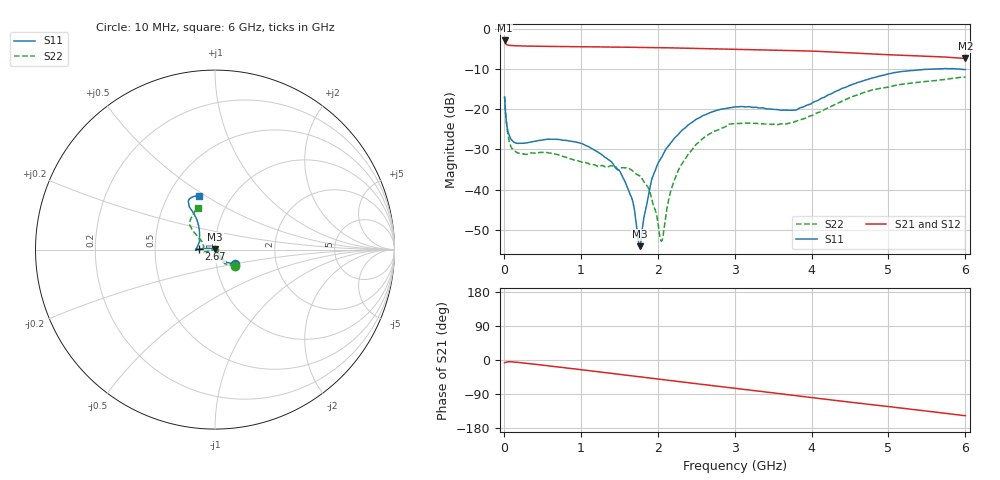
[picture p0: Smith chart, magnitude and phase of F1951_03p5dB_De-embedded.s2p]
! Integrated Device Technology
! Corporate Headquarters
! 6024 Silver Creek Valley Road
! San Jose, CA 95138  USA
! Phone:  1-408-284-8200
! Toll Free:  1-800-223-1366
! Webpage:  http://www.idt.com/
! Timing and RF Division
! 515 Groton Road, Suite 102
! Westford, MA 01886-6024
! Device:  F1951
! Description: 6-bit 0.5 dB Digital Step Attenuator
! Frequency:  100.0 -  4000.00 MHz
! Package:  4x4 mm Thin QFN Plastic Package: 24 pin
! Ports:  2 RF, 6 DC
!  Pin  1  = NC
!  Pin  2  = RF1  =  Port 1
!  Pin  3  = GND
!  Pin  4  = NC
!  Pin  5  = Serial Data Out (SDO)
!  Pin  6  = NC
!  Pin  7  = Reset Bar ( RSTb)
!  Pin  8  = Clock (CLK)
!  Pin  9  = Chip Select Bar (CSb)
!  Pin 10  = NC
!  Pin 11  = Serial Data In (SDI)
!  Pin 12  = NC
!  Pin 13  = NC
!  Pin 14  = VDD
!  Pin 15  = NC
!  Pin 16  = GND
!  Pin 17  = RF2  =  Port 2
!  Pin 18  = NC
!  Pin 19  = GND
!  Pin 20  = GND
!  Pin 21  = GND
!  Pin 22  = GND
!  Pin 23  = GND
!  Pin 24  = GND
! State:  7
! Atten State:  3.5 dB
! Voltage:  +3.30 Volts
! Current:  0.488 mA
! Data:  The device was measured on a F195X evaluation board which has
!  individual transmission lines to the RF pins.  Data was collected
!  de-embedded using a Automatic Fixture Removal [AFR] (Keysight Technologies).
!  The reference plane is the edge of the package pin.
! Misc:  Lot Code  1225BCA
!  Action Tracker AT0399
! Date Measured:  2018-09-13
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# GHz S dB R 50
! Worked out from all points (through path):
!   600 points, 10 MHz to 6 GHz, reference 50 ohm
!   highest |S21| = -2.91 dB at 10 MHz (marker M1); lowest = -7.4 dB at 6 GHz (marker M2)
!   group delay of S21, straight-line fit = 67.5 ps
!   lowest |S11| = -54.0 dB at 1.77 GHz (marker M3), VSWR 1.00, Z = 50.1 + j0.18 ohm
!   |S11| at or under -10 dB: start of sweep to 5.614 GHz; 5.923 GHz to end of sweep
!   |S22| runs from -52.8 to -12.0 dB; largest |S21 - S12| = 0.00078
!   S11 on the Smith chart (normalised r, x): 10 MHz: 1.24, -0.21; 2.67 GHz: 0.84, +0.00; 6 GHz: 0.71, +0.47
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0.01  -17.04 -36.0  -2.91 -6.9  -2.92 -6.9  -16.80 -38.8
0.07  -26.42 -50.7  -4.12 -4.6  -4.12 -4.6  -28.00 -66.2
0.15  -28.35 -54.9  -4.23 -5.7  -4.23 -5.6  -30.47 -70.3
1.01  -28.51 -53.0  -4.49 -25.7  -4.49 -25.7  -33.11 -42.9
1.37  -32.64 -34.1  -4.54 -34.4  -4.55 -34.4  -34.18 -2.3
1.52  -35.85 -22.5  -4.58 -37.9  -4.58 -37.9  -34.59 14.3
1.66  -41.93 -11.4  -4.61 -41.4  -4.61 -41.5  -35.09 20.8
1.74  -51.39 25.5  -4.62 -43.4  -4.63 -43.4  -36.31 24.2
1.77  -54.02 64.4  -4.63 -44.2  -4.63 -44.2  -36.61 26.1
1.89  -40.40 156.8  -4.67 -47.2  -4.67 -47.2  -40.07 35.7
2.01  -33.22 164.7  -4.70 -50.2  -4.70 -50.2  -49.12 72.5
2.04  -32.29 166.0  -4.71 -50.9  -4.71 -50.9  -52.67 106.4
2.06  -31.66 166.0  -4.72 -51.4  -4.72 -51.4  -52.44 130.3
2.16  -28.64 169.7  -4.75 -53.9  -4.75 -53.9  -41.09 -178.6
2.29  -25.75 172.4  -4.79 -57.1  -4.80 -57.2  -34.37 -169.7
2.49  -22.62 176.2  -4.87 -62.1  -4.87 -62.1  -28.94 -166.2
2.67  -20.93 178.9  -4.95 -66.6  -4.96 -66.6  -26.17 -167.1
3.01  -19.40 -178.6  -5.10 -74.8  -5.11 -74.8  -23.56 -172.2
3.76  -20.25 153.0  -5.42 -93.2  -5.43 -93.2  -23.25 159.7
4.01  -18.43 135.7  -5.56 -99.4  -5.56 -99.4  -21.53 149.3
5.01  -11.20 121.0  -6.47 -123.1  -6.47 -123.1  -14.46 136.5
6  -10.15 106.9  -7.39 -146.9  -7.39 -146.9  -11.98 112.1
